| IBIS file stm32f7x2_ufbga176.ibs
[IBIS ver] 4.2
[File name] stm32f7x2_ufbga176.ibs
[File Rev] 1.1
[Date]  21-12-2016
[Source] Data Created at STMicroelectronics
[Notes]  File originated from ELDO simulations.
[Disclaimer]  This information is for modeling purpose only and is
   not guaranted.
   The information is subject to change without notice.
[Copyright] Copyright 2017 STMicroelectronics Inc.
|   Component stm32f7x2_ufbga176
[Component] stm32f7x2_ufbga176
[Manufacturer] STMicroelectronics
[Package]
| variable   typ   min   max
R_pkg   0.0   0.0   0.0
L_pkg   0.0H   0.0H   0.0H
C_pkg   0.0F   0.0F   0.0F
[Pin]  signal_name   model_name   R_pin   L_pin   C_pin
A1 PE3 io8p_arsudq_ft
A10 PB3 io8p_arsudq_ft
A11 PD7 io8p_arsudq_ft
A12 PC12 io8p_arsudq_ft
A13 PA15 io8p_arsudq_ft
A14 PA14 io8p_arsudq_ft
A15 PA13 io8p_arsudq_ft
A2 PE2 io8p_arsudq_ft
A3 PE1 io8p_arsudq_ft
A4 PE0 io8p_arsudq_ft
A5 PB8 io8p_arsudq_i2c_ft
A6 PB5 io8p_ar3wsudq_ft
A7 PG14 io8p_arsudq_ft
A8 PG13 io8p_arsudq_ft
A9 PB4 io8p_arsudq_ft
B1 PE4 io8p_arsudq_ft
B10 PG10 io8p_arsudq_ft
B11 PD6 io8p_arsudq_ft
B12 PD0 io8p_arsudq_ft
B13 PC11 io8p_arsudq_ft
B14 PC10 io8p_arsudq_ft
B15 PA12 io8usb_lsfs_otg_ft
B2 PE5 io8p_arsudq_ft
B3 PE6 io8p_arsudq_ft
B4 PB9 io8p_arsudq_i2c_ft
B5 PB7 io8p_arsudq_i2c_ft
B6 PB6 io8p_arsudq_i2c_ft
B7 PG15 io8p_arsudq_ft
B8 PG12 io8p_arsudq_ft
B9 PG11 io8p_arsudq_ft
C1 VBAT power
C10 PG9 io8p_arsudq_ft
C11 PD5 io8p_arsudq_ft
C12 PD1 io8p_arsudq_ft
C13 PI3 io8p_arsudq_ft
C14 PI2 io8p_arsudq_ft
C15 PA11 io8usb_lsfs_otg_ft
C2 PI7 io8p_arsudq_ft
C3 PI6 io8p_arsudq_ft
C4 PI5 io8p_arsudq_ft
C5 VDD power
C6 PDR_ON gnd
C7 VDD power
C8 VDDSDMMC power
C9 VDD power
D1 PC13 io8p_arwsudq_ft_v33
D10 PD4 io8p_arsudq_ft
D11 PD3 io8p_arsudq_ft
D12 PD2 io8p_arsudq_ft
D13 PH15 io8p_arsudq_ft
D14 PI1 io8p_arsudq_ft
D15 PA10 io8usb_id_otg_ft
D2 PI8 io8p_arsudq_ft_v33
D3 PI9 io8p_arsudq_ft
D4 PI4 io8p_arsudq_ft
D5 VSS gnd
D6 BOOT0 vpp_test_hv
D7 VSS gnd
D8 VSS gnd
D9 VSS gnd
E1 PC14-OSC32_IN io8p_arwsudq_ft_v33
E12 PH13 io8p_arsudq_ft
E13 PH14 io8p_arsudq_ft
E14 PI0 io8p_arsudq_ft
E15 PA9 io8usb_vbus_otg_ft
E2 PF0 io8p_arsudq_i2c_ft
E3 PI10 io8p_arsudq_ft
E4 PI11 io8p_arsudq_ft_v33
F1 PC15-OSC32_OUT io8p_arwsudq_ft
F12 VSS gnd
F13 VCAP_2 power
F14 PC9 io8p_arsudq_i2c_ft
F15 PA8 io8p_arsudq_i2c_ft
F2 VSS gnd
F3 VDD power
F4 PH2 io8p_arsudq_ft
F6 VSS gnd
F7 VSS gnd
F8 VSS gnd
F9 VSS gnd
F10 VSS gnd
G1 PH0-OSC_IN io8p_arsudq_ft
G12 VSS gnd
G13 VDD power
G14 PC8 io8p_arsudq_ft
G15 PC7 io8p_arsudq_ft
G2 VSS gnd
G3 VDD power
G4 PH3 io8p_arsudq_ft
G6 VSS gnd
G7 VSS gnd
G8 VSS gnd
G9 VSS gnd
G10 VSS gnd
H1 PH1-OSC_OUT io8p_arsudq_ft
H12 VSS gnd
H13 VDDUSB power
H14 PG8 io8p_arsudq_ft
H15 PC6 io8p_arsudq_ft
H2 PF2 io8p_arsudq_ft
H3 PF1 io8p_arsudq_i2c_ft
H4 PH4 io8p_arsudq_i2c_ft
H6 VSS gnd
H7 VSS gnd
H8 VSS gnd
H9 VSS gnd
H10 VSS gnd
J1 NRST ioreset_ft_v33
J12 VDD power
J13 VDD power
J14 PG7 io8p_arsudq_ft
J15 PG6 io8p_arsudq_ft
J2 PF3 io8p_arwsudq_ft
J3 PF4 io8p_arwsudq_ft
J4 PH5 io8p_arsudq_i2c_ft
J6 VSS gnd
J7 VSS gnd
J8 VSS gnd
J9 VSS gnd
J10 VSS gnd
K1 PF7 io8p_arwsudq_ft
K12 PH12 io8p_arsudq_ft
K13 PG5 io8p_arsudq_ft
K14 PG4 io8p_arsudq_ft
K15 PG3 io8p_arsudq_ft
K2 PF6 io8p_arwsudq_ft
K3 PF5 io8p_arwsudq_ft
K4 VDD power
K6 VSS gnd
K7 VSS gnd
K8 VSS gnd
K9 VSS gnd
K10 VSS gnd
L1 PF10 io8p_arwsudq_ft
L12 PH11 io8p_arsudq_ft
L13 PH10 io8p_arsudq_ft
L14 PD15 io8p_arsudq_ft
L15 PG2 io8p_arsudq_ft
L2 PF9 io8p_arwsudq_ft
L3 PF8 io8p_arwsudq_ft
L4 BYPASS_REG gnd
M1 VSSA gnd
M10 VCAP_1 power
M11 PH6 io8p_arsudq_ft
M12 PH8 io8p_arsudq_i2c_ft
M13 PH9 io8p_arsudq_ft
M14 PD14 io8p_arsudq_ft
M15 PD13 io8p_arsudq_ft
M2 PC0 io8p_ar3wsudq_ft
M3 PC1 io8p_ar3wsudq_ft_v33
M4 PC2 io8p_ar3wsudq_ft
M5 PC3 io8p_ar3wsudq_ft
M6 PB2 io8p_ar3wsudq_ft
M7 PG1 io8p_arsudq_ft
M8 VSS gnd
M9 VSS gnd
N1 VREF- gnd
N10 VDD power
N11 PE13 io8p_arsudq_ft
N12 PH7 io8p_arsudq_i2c_ft
N13 PD12 io8p_arsudq_ft
N14 PD11 io8p_arsudq_ft
N15 PD10 io8p_arsudq_ft
N2 PA1 io8p_ar3wsudq_ft
N3 PA0-WKUP io8p_ar3wsudq_ft_v33
N4 PA4 io8p_ar3wsudq_ft
N5 PC4 io8p_ar3wsudq_ft
N6 PF13 io8p_arsudq_ft
N7 PG0 io8p_arsudq_ft
N8 VDD power
N9 VDD power
P1 VREF+ power
P10 PE11 io8p_arsudq_ft
P11 PE14 io8p_arsudq_ft
P12 PB12 io8usb_id_otg_ft
P13 PB13 io8usb_vbus_otg_ft
P14 PD9 io8p_arsudq_ft
P15 PD8 io8p_arsudq_ft
P2 PA2 io8p_ar3wsudq_ft_v33
P3 PA6 io8p_ar3wsudq_ft
P4 PA5 io8p_ar3wsudq_ft
P5 PC5 io8p_ar3wsudq_ft
P6 PF12 io8p_arsudq_ft
P7 PF15 io8p_arsudq_ft
P8 PE8 io8p_arsudq_ft
P9 PE9 io8p_arsudq_ft
R1 VDDA power
R10 PE12 io8p_arsudq_ft
R11 PE15 io8p_ar3wsudq_ft
R12 PB10 io8p_arsudq_i2c_ft
R13 PB11 io8p_arsudq_i2c_ft
R14 PB14 io8usb_lsfs_otg_ft
R15 PB15 io8usb_lsfs_otg_ft
R2 PA3 io8p_ar3wsudq_ft
R3 PA7 io8p_ar3wsudq_ft
R4 PB1 io8p_ar3wsudq_ft
R5 PB0 io8p_ar3wsudq_ft
R6 PF11 io8p_arsudq_ft
R7 PF14 io8p_arsudq_ft
R8 PE7 io8p_arsudq_ft
R9 PE10 io8p_arsudq_ft
[Diff Pin]   inv_pin   vdiff   tdelay_typ  tdelay_min  tdelay_max
B15   C15   NA   NA   NA   NA
R14   R15   NA   NA   NA   NA
[Model Selector] io8p_ar3wsudq_ft
io8p00_ar3wsudq_ft_pd_lv  "SPEED00 1P8V, PD=40kOhm"
io8p00_ar3wsudq_ft_pu_lv  "SPEED00 1P8V, PU=40kOhm"
io8p00_ar3wsudq_ft_lv  "SPEED00 1P8V"
io8p01_ar3wsudq_ft_pd_lv  "SPEED01 1P8V, PD=40kOhm"
io8p01_ar3wsudq_ft_pu_lv  "SPEED01 1P8V, PU=40kOhm"
io8p01_ar3wsudq_ft_lv  "SPEED01 1P8V"
io8p10_ar3wsudq_ft_pd_lv  "SPEED10 1P8V, PD=40kOhm"
io8p10_ar3wsudq_ft_pu_lv  "SPEED10 1P8V, PU=40kOhm"
io8p10_ar3wsudq_ft_lv  "SPEED10 1P8V"
io8p11_ar3wsudq_ft_pd_lv  "SPEED11 1P8V, PD=40kOhm"
io8p11_ar3wsudq_ft_pu_lv  "SPEED11 1P8V, PU=40kOhm"
io8p11_ar3wsudq_ft_lv  "SPEED11 1P8V"
io8p00_ar3wsudq_ft_pd  "SPEED00, PD=40kOhm"
io8p00_ar3wsudq_ft_pu  "SPEED00, PU=40kOhm"
io8p00_ar3wsudq_ft  "SPEED00"
io8p01_ar3wsudq_ft_pd  "SPEED01, PD=40kOhm"
io8p01_ar3wsudq_ft_pu  "SPEED01, PU=40kOhm"
io8p01_ar3wsudq_ft  "SPEED01"
io8p10_ar3wsudq_ft_pd  "SPEED10, PD=40kOhm"
io8p10_ar3wsudq_ft_pu  "SPEED10, PU=40kOhm"
io8p10_ar3wsudq_ft  "SPEED10"
io8p11_ar3wsudq_ft_pd  "SPEED11, PD=40kOhm"
io8p11_ar3wsudq_ft_pu  "SPEED11, PU=40kOhm"
io8p11_ar3wsudq_ft  "SPEED11"
[Model Selector] io8p_ar3wsudq_ft_v33
io8p00_ar3wsudq_ft_v33_pd_lv  "SPEED00 1P8V, PD=40kOhm"
io8p00_ar3wsudq_ft_v33_pu_lv  "SPEED00 1P8V, PU=40kOhm"
io8p00_ar3wsudq_ft_v33_lv  "SPEED00 1P8V"
io8p01_ar3wsudq_ft_v33_pd_lv  "SPEED01 1P8V, PD=40kOhm"
io8p01_ar3wsudq_ft_v33_pu_lv  "SPEED01 1P8V, PU=40kOhm"
io8p01_ar3wsudq_ft_v33_lv  "SPEED01 1P8V"
io8p10_ar3wsudq_ft_v33_pd_lv  "SPEED10 1P8V, PD=40kOhm"
io8p10_ar3wsudq_ft_v33_pu_lv  "SPEED10 1P8V, PU=40kOhm"
io8p10_ar3wsudq_ft_v33_lv  "SPEED10 1P8V"
io8p11_ar3wsudq_ft_v33_pd_lv  "SPEED11 1P8V, PD=40kOhm"
io8p11_ar3wsudq_ft_v33_pu_lv  "SPEED11 1P8V, PU=40kOhm"
io8p11_ar3wsudq_ft_v33_lv  "SPEED11 1P8V"
io8p00_ar3wsudq_ft_v33_pd  "SPEED00, PD=40kOhm"
io8p00_ar3wsudq_ft_v33_pu  "SPEED00, PU=40kOhm"
io8p00_ar3wsudq_ft_v33  "SPEED00"
io8p01_ar3wsudq_ft_v33_pd  "SPEED01, PD=40kOhm"
io8p01_ar3wsudq_ft_v33_pu  "SPEED01, PU=40kOhm"
io8p01_ar3wsudq_ft_v33  "SPEED01"
io8p10_ar3wsudq_ft_v33_pd  "SPEED10, PD=40kOhm"
io8p10_ar3wsudq_ft_v33_pu  "SPEED10, PU=40kOhm"
io8p10_ar3wsudq_ft_v33  "SPEED10"
io8p11_ar3wsudq_ft_v33_pd  "SPEED11, PD=40kOhm"
io8p11_ar3wsudq_ft_v33_pu  "SPEED11, PU=40kOhm"
io8p11_ar3wsudq_ft_v33  "SPEED11"
[Model Selector] io8p_arsudq_ft
io8p00_arsudq_ft_pd_lv  "SPEED00 1P8V, PD=40kOhm"
io8p00_arsudq_ft_pu_lv  "SPEED00 1P8V, PU=40kOhm"
io8p00_arsudq_ft_lv  "SPEED00 1P8V"
io8p01_arsudq_ft_pd_lv  "SPEED01 1P8V, PD=40kOhm"
io8p01_arsudq_ft_pu_lv  "SPEED01 1P8V, PU=40kOhm"
io8p01_arsudq_ft_lv  "SPEED01 1P8V"
io8p10_arsudq_ft_pd_lv  "SPEED10 1P8V, PD=40kOhm"
io8p10_arsudq_ft_pu_lv  "SPEED10 1P8V, PU=40kOhm"
io8p10_arsudq_ft_lv  "SPEED10 1P8V"
io8p11_arsudq_ft_pd_lv  "SPEED11 1P8V, PD=40kOhm"
io8p11_arsudq_ft_pu_lv  "SPEED11 1P8V, PU=40kOhm"
io8p11_arsudq_ft_lv  "SPEED11 1P8V"
io8p00_arsudq_ft_pd  "SPEED00, PD=40kOhm"
io8p00_arsudq_ft_pu  "SPEED00, PU=40kOhm"
io8p00_arsudq_ft  "SPEED00"
io8p01_arsudq_ft_pd  "SPEED01, PD=40kOhm"
io8p01_arsudq_ft_pu  "SPEED01, PU=40kOhm"
io8p01_arsudq_ft  "SPEED01"
io8p10_arsudq_ft_pd  "SPEED10, PD=40kOhm"
io8p10_arsudq_ft_pu  "SPEED10, PU=40kOhm"
io8p10_arsudq_ft  "SPEED10"
io8p11_arsudq_ft_pd  "SPEED11, PD=40kOhm"
io8p11_arsudq_ft_pu  "SPEED11, PU=40kOhm"
io8p11_arsudq_ft  "SPEED11"
[Model Selector] io8p_arsudq_i2c_ft
io8prog_1v8_i2c_pd  "5V Tol GPIO 1.8V range i2c functionality with pull down"
io8prog_1v8_i2c_pu  "5V Tol GPIO 1.8V range i2c functionality with pull up"
io8prog_1v8_i2c  "5V Tol GPIO 1.8V range i2c functionality"
io8prog_3v3_i2c_pd  "5V Tol GPIO 3.3V range i2c functionality with pull down"
io8prog_3v3_i2c_pu  "5V Tol GPIO 3.3V range i2c functionality with pull up"
io8prog_3v3_i2c  "5V Tol GPIO 3.3V range i2c functionality"
io8prog_1v8_pd_00  "5V Tol GPIO 1.8V range with pd speed 00"
io8prog_1v8_pu_00  "5V Tol GPIO 1.8V range with pu speed 00"
io8prog_1v8_00  "5V Tol GPIO 1.8V range speed 00"
io8prog_3v3_pd_00  "5V Tol GPIO 3.3V range with pd speed 00"
io8prog_3v3_pu_00  "5V Tol GPIO 3.3V range with pu speed 00"
io8prog_3v3_00  "5V Tol GPIO 3.3V range speed 00"
io8prog_1v8_pd_01  "5V Tol GPIO 1.8V range with pd speed 01"
io8prog_1v8_pu_01  "5V Tol GPIO 1.8V range with pu speed 01"
io8prog_1v8_01  "5V Tol GPIO 1.8V range speed 01"
io8prog_3v3_pd_01  "5V Tol GPIO 3.3V range with pd speed 01"
io8prog_3v3_pu_01  "5V Tol GPIO 3.3V range with pu speed 01"
io8prog_3v3_01  "5V Tol GPIO 3.3V range speed 01"
io8prog_1v8_pd_10  "5V Tol GPIO 1.8V range with pd speed 10"
io8prog_1v8_pu_10  "5V Tol GPIO 1.8V range with pu speed 10"
io8prog_1v8_10  "5V Tol GPIO 1.8V range speed 10"
io8prog_3v3_pd_10  "5V Tol GPIO 3.3V range with pd speed 10"
io8prog_3v3_pu_10  "5V Tol GPIO 3.3V range with pu speed 10"
io8prog_3v3_10  "5V Tol GPIO 3.3V range speed 10"
io8prog_1v8_pd_11  "5V Tol GPIO 1.8V range with pd speed 11"
io8prog_1v8_pu_11  "5V Tol GPIO 1.8V range with pu speed 11"
io8prog_1v8_11  "5V Tol GPIO 1.8V range speed 11"
io8prog_3v3_pd_11  "5V Tol GPIO 3.3V range with pd speed 11"
io8prog_3v3_pu_11  "5V Tol GPIO 3.3V range with pu speed 11"
io8prog_3v3_11  "5V Tol GPIO 3.3V range speed 11"
[Model Selector] io8p_arwsudq_ft
io8p00_arwsudq_ft_pd_lv  "SPEED00 1P8V, PD=40kOhm"
io8p00_arwsudq_ft_pu_lv  "SPEED00 1P8V, PU=40kOhm"
io8p00_arwsudq_ft_lv  "SPEED00 1P8V"
io8p01_arwsudq_ft_pd_lv  "SPEED01 1P8V, PD=40kOhm"
io8p01_arwsudq_ft_pu_lv  "SPEED01 1P8V, PU=40kOhm"
io8p01_arwsudq_ft_lv  "SPEED01 1P8V"
io8p10_arwsudq_ft_pd_lv  "SPEED10 1P8V, PD=40kOhm"
io8p10_arwsudq_ft_pu_lv  "SPEED10 1P8V, PU=40kOhm"
io8p10_arwsudq_ft_lv  "SPEED10 1P8V"
io8p11_arwsudq_ft_pd_lv  "SPEED11 1P8V, PD=40kOhm"
io8p11_arwsudq_ft_pu_lv  "SPEED11 1P8V, PU=40kOhm"
io8p11_arwsudq_ft_lv  "SPEED11 1P8V"
io8p00_arwsudq_ft_pd  "SPEED00, PD=40kOhm"
io8p00_arwsudq_ft_pu  "SPEED00, PU=40kOhm"
io8p00_arwsudq_ft  "SPEED00"
io8p01_arwsudq_ft_pd  "SPEED01, PD=40kOhm"
io8p01_arwsudq_ft_pu  "SPEED01, PU=40kOhm"
io8p01_arwsudq_ft  "SPEED01"
io8p10_arwsudq_ft_pd  "SPEED10, PD=40kOhm"
io8p10_arwsudq_ft_pu  "SPEED10, PU=40kOhm"
io8p10_arwsudq_ft  "SPEED10"
io8p11_arwsudq_ft_pd  "SPEED11, PD=40kOhm"
io8p11_arwsudq_ft_pu  "SPEED11, PU=40kOhm"
io8p11_arwsudq_ft  "SPEED11"
[Model Selector] io8p_arwsudq_ft_v33
io8p00_arwsudq_ft_v33_pd_lv  "SPEED00 1P8V, PD=40kOhm"
io8p00_arwsudq_ft_v33_pu_lv  "SPEED00 1P8V, PU=40kOhm"
io8p00_arwsudq_ft_v33_lv  "SPEED00 1P8V"
io8p01_arwsudq_ft_v33_pd_lv  "SPEED01 1P8V, PD=40kOhm"
io8p01_arwsudq_ft_v33_pu_lv  "SPEED01 1P8V, PU=40kOhm"
io8p01_arwsudq_ft_v33_lv  "SPEED01 1P8V"
io8p10_arwsudq_ft_v33_pd_lv  "SPEED10 1P8V, PD=40kOhm"
io8p10_arwsudq_ft_v33_pu_lv  "SPEED10 1P8V, PU=40kOhm"
io8p10_arwsudq_ft_v33_lv  "SPEED10 1P8V"
io8p11_arwsudq_ft_v33_pd_lv  "SPEED11 1P8V, PD=40kOhm"
io8p11_arwsudq_ft_v33_pu_lv  "SPEED11 1P8V, PU=40kOhm"
io8p11_arwsudq_ft_v33_lv  "SPEED11 1P8V"
io8p00_arwsudq_ft_v33_pd  "SPEED00, PD=40kOhm"
io8p00_arwsudq_ft_v33_pu  "SPEED00, PU=40kOhm"
io8p00_arwsudq_ft_v33  "SPEED00"
io8p01_arwsudq_ft_v33_pd  "SPEED01, PD=40kOhm"
io8p01_arwsudq_ft_v33_pu  "SPEED01, PU=40kOhm"
io8p01_arwsudq_ft_v33  "SPEED01"
io8p10_arwsudq_ft_v33_pd  "SPEED10, PD=40kOhm"
io8p10_arwsudq_ft_v33_pu  "SPEED10, PU=40kOhm"
io8p10_arwsudq_ft_v33  "SPEED10"
io8p11_arwsudq_ft_v33_pd  "SPEED11, PD=40kOhm"
io8p11_arwsudq_ft_v33_pu  "SPEED11, PU=40kOhm"
io8p11_arwsudq_ft_v33  "SPEED11"
[Model Selector] io8p_arsudq_ft_v33
io8p00_arsudq_ft_v33_pd_lv  "SPEED00 1P8V, PD=40kOhm"
io8p00_arsudq_ft_v33_pu_lv  "SPEED00 1P8V, PU=40kOhm"
io8p00_arsudq_ft_v33_lv  "SPEED00 1P8V"
io8p01_arsudq_ft_v33_pd_lv  "SPEED01 1P8V, PD=40kOhm"
io8p01_arsudq_ft_v33_pu_lv  "SPEED01 1P8V, PU=40kOhm"
io8p01_arsudq_ft_v33_lv  "SPEED01 1P8V"
io8p10_arsudq_ft_v33_pd_lv  "SPEED10 1P8V, PD=40kOhm"
io8p10_arsudq_ft_v33_pu_lv  "SPEED10 1P8V, PU=40kOhm"
io8p10_arsudq_ft_v33_lv  "SPEED10 1P8V"
io8p11_arsudq_ft_v33_pd_lv  "SPEED11 1P8V, PD=40kOhm"
io8p11_arsudq_ft_v33_pu_lv  "SPEED11 1P8V, PU=40kOhm"
io8p11_arsudq_ft_v33_lv  "SPEED11 1P8V"
io8p00_arsudq_ft_v33_pd  "SPEED00, PD=40kOhm"
io8p00_arsudq_ft_v33_pu  "SPEED00, PU=40kOhm"
io8p00_arsudq_ft_v33  "SPEED00"
io8p01_arsudq_ft_v33_pd  "SPEED01, PD=40kOhm"
io8p01_arsudq_ft_v33_pu  "SPEED01, PU=40kOhm"
io8p01_arsudq_ft_v33  "SPEED01"
io8p10_arsudq_ft_v33_pd  "SPEED10, PD=40kOhm"
io8p10_arsudq_ft_v33_pu  "SPEED10, PU=40kOhm"
io8p10_arsudq_ft_v33  "SPEED10"
io8p11_arsudq_ft_v33_pd  "SPEED11, PD=40kOhm"
io8p11_arsudq_ft_v33_pu  "SPEED11, PU=40kOhm"
io8p11_arsudq_ft_v33  "SPEED11"
[Model Selector] io8usb_id_otg_ft
io8p00_id_otg_ft_pd_lv  "SPEED00 1P8V, PD=14kOhm"
io8p00_id_otg_ft_pu_lv  "SPEED00 1P8V, PU=14kOhm"
io8p00_id_otg_ft_lv  "SPEED00 1P8V"
io8p01_id_otg_ft_pd_lv  "SPEED01 1P8V, PD=14kOhm"
io8p01_id_otg_ft_pu_lv  "SPEED01 1P8V, PU=14kOhm"
io8p01_id_otg_ft_lv  "SPEED01 1P8V"
io8p10_id_otg_ft_pd_lv  "SPEED10 1P8V, PD=14kOhm"
io8p10_id_otg_ft_pu_lv  "SPEED10 1P8V, PU=14kOhm"
io8p10_id_otg_ft_lv  "SPEED10 1P8V"
io8p11_id_otg_ft_pd_lv  "SPEED11 1P8V, PD=14kOhm"
io8p11_id_otg_ft_pu_lv  "SPEED11 1P8V, PU=14kOhm"
io8p11_id_otg_ft_lv  "SPEED11 1P8V"
io8p00_id_otg_ft_pd  "SPEED00, PD=14kOhm"
io8p00_id_otg_ft_pu  "SPEED00, PU=14kOhm"
io8p00_id_otg_ft  "SPEED00"
io8p01_id_otg_ft_pd  "SPEED01, PD=14kOhm"
io8p01_id_otg_ft_pu  "SPEED01, PU=14kOhm"
io8p01_id_otg_ft  "SPEED01"
io8p10_id_otg_ft_pd  "SPEED10, PD=14kOhm"
io8p10_id_otg_ft_pu  "SPEED10, PU=14kOhm"
io8p10_id_otg_ft  "SPEED10"
io8p11_id_otg_ft_pd  "SPEED11, PD=14kOhm"
io8p11_id_otg_ft_pu  "SPEED11, PU=14kOhm"
io8p11_id_otg_ft  "SPEED11"
[Model Selector] io8usb_lsfs_otg_ft
io8usb_ls_otg_ft_dpdn_pd  "LS USB DP/DN IO + PD=20kOhm"
io8usb_ls_otg_ft_dpdn_pupu2  "LS USB DP/DN IO + PU/PU2=2.2kOhm"
io8usb_ls_otg_ft_dpdn_pu2  "LS USB DP/DN IO + PU2=1.2kOhm"
io8usb_ls_otg_ft_dpdn_pu  "LS USB DP/DN IO + PU=1.2kOhm"
io8usb_ls_otg_ft_dpdn  "LS USB DP/DN IO"
io8usb_fs_otg_ft_dpdn_pd  "HS USB DP/DN IO + PD=20kOhm"
io8usb_fs_otg_ft_dpdn_pupu2  "HS USB DP/DN IO + PU/PU2=2.2kOhm"
io8usb_fs_otg_ft_dpdn_pu2  "HS USB DP/DN IO + PU2=1.2kOhm"
io8usb_fs_otg_ft_dpdn_pu  "HS USB DP/DN IO + PU=1.2kOhm"
io8usb_fs_otg_ft_dpdn  "HS USB DP/DN IO"
io8p00_lsfs_otg_ft_pd_lv  "SPEED00 1P8V, PD=40kOhm"
io8p00_lsfs_otg_ft_pu_lv  "SPEED00 1P8V, PU=40kOhm"
io8p00_lsfs_otg_ft_lv  "SPEED00 1P8V"
io8p01_lsfs_otg_ft_pd_lv  "SPEED01 1P8V, PD=40kOhm"
io8p01_lsfs_otg_ft_pu_lv  "SPEED01 1P8V, PU=40kOhm"
io8p01_lsfs_otg_ft_lv  "SPEED01 1P8V"
io8p10_lsfs_otg_ft_pd_lv  "SPEED10 1P8V, PD=40kOhm"
io8p10_lsfs_otg_ft_pu_lv  "SPEED10 1P8V, PU=40kOhm"
io8p10_lsfs_otg_ft_lv  "SPEED10 1P8V"
io8p11_lsfs_otg_ft_pd_lv  "SPEED11 1P8V, PD=40kOhm"
io8p11_lsfs_otg_ft_pu_lv  "SPEED11 1P8V, PU=40kOhm"
io8p11_lsfs_otg_ft_lv  "SPEED11 1P8V"
io8p00_lsfs_otg_ft_pd  "SPEED00, PD=40kOhm"
io8p00_lsfs_otg_ft_pu  "SPEED00, PU=40kOhm"
io8p00_lsfs_otg_ft  "SPEED00"
io8p01_lsfs_otg_ft_pd  "SPEED01, PD=40kOhm"
io8p01_lsfs_otg_ft_pu  "SPEED01, PU=40kOhm"
io8p01_lsfs_otg_ft  "SPEED01"
io8p10_lsfs_otg_ft_pd  "SPEED10, PD=40kOhm"
io8p10_lsfs_otg_ft_pu  "SPEED10, PU=40kOhm"
io8p10_lsfs_otg_ft  "SPEED10"
io8p11_lsfs_otg_ft_pd  "SPEED11, PD=40kOhm"
io8p11_lsfs_otg_ft_pu  "SPEED11, PU=40kOhm"
io8p11_lsfs_otg_ft  "SPEED11"
[Model Selector] io8usb_vbus_otg_ft
io8psenb_vbus_otg_ft  "VBUS PULSE, SENSE VB"
io8psenab_vbus_otg_ft  "VBUS PULSE, SENSE VA and VB"
io8psena_vbus_otg_ft  "VBUS PULSE, SENSE VA"
io8psen_vbus_otg_ft  "VBUS PULSE"
io8p00_vbus_otg_ft_pd_lv  "SPEED00 1P8V, PD=40kOhm"
io8p00_vbus_otg_ft_pu_lv  "SPEED00 1P8V, PU=40kOhm"
io8p00_vbus_otg_ft_lv  "SPEED00 1P8V"
io8p01_vbus_otg_ft_pd_lv  "SPEED01 1P8V, PD=40kOhm"
io8p01_vbus_otg_ft_pu_lv  "SPEED01 1P8V, PU=40kOhm"
io8p01_vbus_otg_ft_lv  "SPEED01 1P8V"
io8p10_vbus_otg_ft_pd_lv  "SPEED10 1P8V, PD=40kOhm"
io8p10_vbus_otg_ft_pu_lv  "SPEED10 1P8V, PU=40kOhm"
io8p10_vbus_otg_ft_lv  "SPEED10 1P8V"
io8p11_vbus_otg_ft_pd_lv  "SPEED11 1P8V, PD=40kOhm"
io8p11_vbus_otg_ft_pu_lv  "SPEED11 1P8V, PU=40kOhm"
io8p11_vbus_otg_ft_lv  "SPEED11 1P8V"
io8p00_vbus_otg_ft_pd  "SPEED00, PD=40kOhm"
io8p00_vbus_otg_ft_pu  "SPEED00, PU=40kOhm"
io8p00_vbus_otg_ft  "SPEED00"
io8p01_vbus_otg_ft_pd  "SPEED01, PD=40kOhm"
io8p01_vbus_otg_ft_pu  "SPEED01, PU=40kOhm"
io8p01_vbus_otg_ft  "SPEED01"
io8p10_vbus_otg_ft_pd  "SPEED10, PD=40kOhm"
io8p10_vbus_otg_ft_pu  "SPEED10, PU=40kOhm"
io8p10_vbus_otg_ft  "SPEED10"
io8p11_vbus_otg_ft_pd  "SPEED11, PD=40kOhm"
io8p11_vbus_otg_ft_pu  "SPEED11, PU=40kOhm"
io8p11_vbus_otg_ft  "SPEED11"
[Model Selector] ioreset_ft_v33
ioreset_ft_v33_pu_lv  "IORESET 1P8V + PU=40kOhm"
ioreset_ft_v33_nopu_lv  "IORESET 1P8V"
ioreset_ft_v33_pu  "IORESET + PU=40kOhm"
ioreset_ft_v33_nopu  "IORESET"
[Model Selector] vpp_test_hv
vpp_test_hv_2p4  "Input Buffer 1P8V"
vpp_test_hv_3p3  "Input Buffer"
| Models and submodels in the file (266): io8p00_ar3wsudq_ft_pd_lv (I/O), io8p00_ar3wsudq_ft_pu_lv (I/O), io8p00_ar3wsudq_ft_lv (I/O), io8p01_ar3wsudq_ft_pd_lv (I/O), io8p01_ar3wsudq_ft_pu_lv (I/O), io8p01_ar3wsudq_ft_lv (I/O), io8p10_ar3wsudq_ft_pd_lv (I/O), io8p10_ar3wsudq_ft_pu_lv (I/O), io8p10_ar3wsudq_ft_lv (I/O), io8p11_ar3wsudq_ft_pd_lv (I/O), io8p11_ar3wsudq_ft_pu_lv (I/O), io8p11_ar3wsudq_ft_lv (I/O), io8p00_ar3wsudq_ft_pd (I/O), io8p00_ar3wsudq_ft_pu (I/O), io8p00_ar3wsudq_ft (I/O), io8p01_ar3wsudq_ft_pd (I/O), io8p01_ar3wsudq_ft_pu (I/O), io8p01_ar3wsudq_ft (I/O), io8p10_ar3wsudq_ft_pd (I/O), io8p10_ar3wsudq_ft_pu (I/O), io8p10_ar3wsudq_ft (I/O), io8p11_ar3wsudq_ft_pd (I/O), io8p11_ar3wsudq_ft_pu (I/O), io8p11_ar3wsudq_ft (I/O), io8p00_ar3wsudq_ft_v33_pd_lv (I/O), io8p00_ar3wsudq_ft_v33_pu_lv (I/O), io8p00_ar3wsudq_ft_v33_lv (I/O), io8p01_ar3wsudq_ft_v33_pd_lv (I/O), io8p01_ar3wsudq_ft_v33_pu_lv (I/O), io8p01_ar3wsudq_ft_v33_lv (I/O), io8p10_ar3wsudq_ft_v33_pd_lv (I/O), io8p10_ar3wsudq_ft_v33_pu_lv (I/O), io8p10_ar3wsudq_ft_v33_lv (I/O), io8p11_ar3wsudq_ft_v33_pd_lv (I/O), io8p11_ar3wsudq_ft_v33_pu_lv (I/O), io8p11_ar3wsudq_ft_v33_lv (I/O), io8p00_ar3wsudq_ft_v33_pd (I/O), io8p00_ar3wsudq_ft_v33_pu (I/O), io8p00_ar3wsudq_ft_v33 (I/O), io8p01_ar3wsudq_ft_v33_pd (I/O), io8p01_ar3wsudq_ft_v33_pu (I/O), io8p01_ar3wsudq_ft_v33 (I/O), io8p10_ar3wsudq_ft_v33_pd (I/O), io8p10_ar3wsudq_ft_v33_pu (I/O), io8p10_ar3wsudq_ft_v33 (I/O), io8p11_ar3wsudq_ft_v33_pd (I/O), io8p11_ar3wsudq_ft_v33_pu (I/O), io8p11_ar3wsudq_ft_v33 (I/O), io8p00_arsudq_ft_pd_lv (I/O), io8p00_arsudq_ft_pu_lv (I/O), io8p00_arsudq_ft_lv (I/O), io8p01_arsudq_ft_pd_lv (I/O), io8p01_arsudq_ft_pu_lv (I/O), io8p01_arsudq_ft_lv (I/O), io8p10_arsudq_ft_pd_lv (I/O), io8p10_arsudq_ft_pu_lv (I/O), io8p10_arsudq_ft_lv (I/O), io8p11_arsudq_ft_pd_lv (I/O), io8p11_arsudq_ft_pu_lv (I/O), io8p11_arsudq_ft_lv (I/O), io8p00_arsudq_ft_pd (I/O), io8p00_arsudq_ft_pu (I/O), io8p00_arsudq_ft (I/O), io8p01_arsudq_ft_pd (I/O), io8p01_arsudq_ft_pu (I/O), io8p01_arsudq_ft (I/O), io8p10_arsudq_ft_pd (I/O), io8p10_arsudq_ft_pu (I/O), io8p10_arsudq_ft (I/O), io8p11_arsudq_ft_pd (I/O), io8p11_arsudq_ft_pu (I/O), io8p11_arsudq_ft (I/O), io8prog_1v8_i2c_pd (I/O), io8prog_1v8_i2c_pu (I/O), io8prog_1v8_i2c (I/O), io8prog_3v3_i2c_pd (I/O), io8prog_3v3_i2c_pu (I/O), io8prog_3v3_i2c (I/O), io8prog_1v8_pd_00 (I/O), io8prog_1v8_pu_00 (I/O)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
